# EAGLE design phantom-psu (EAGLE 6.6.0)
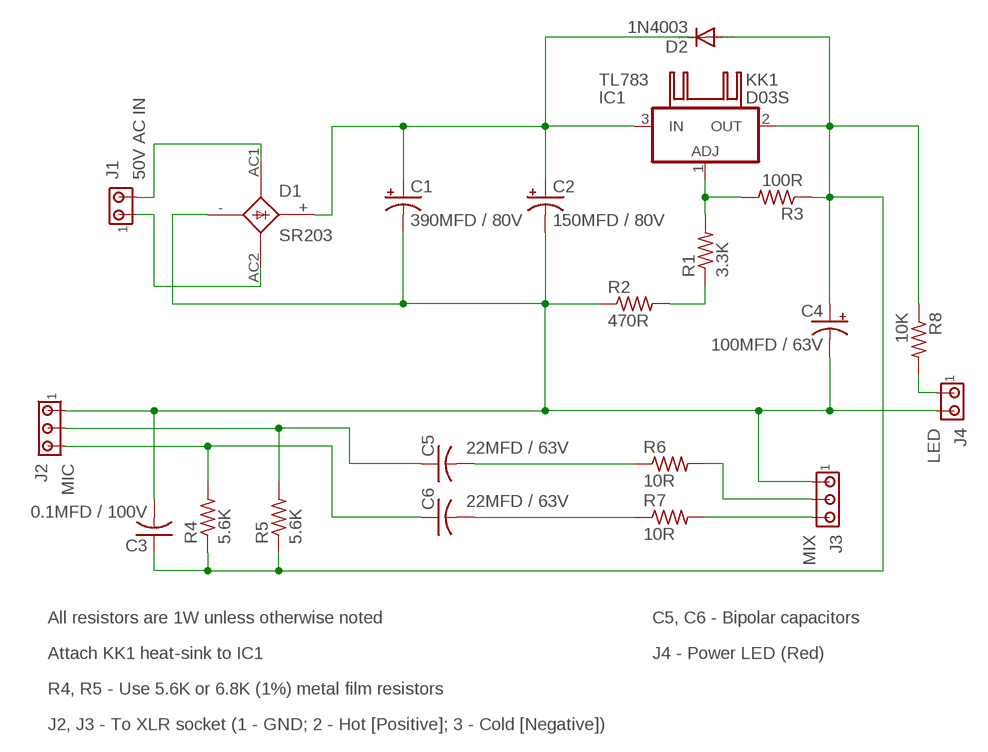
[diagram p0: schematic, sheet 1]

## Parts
C1  390MFD / 80V  CPOL-USE5-10.5  [E5-10,5]
C2  150MFD / 80V  CPOL-USE5-10.5  [E5-10,5]
C3  0.1MFD / 100V  C-US075-063X106  [C075-063X106]
C4  100MFD / 63V  CPOL-USE3.5-8  [E3,5-8]
C5  22MFD / 63V  NON-POL_CAP  [CAP]
C6  22MFD / 63V  NON-POL_CAP  [CAP]
D1  SR203  RS203  [RS-2]
D2  1N4003  1N4004  [DO41-10]
IC1  TL783  [TO220V]
J1  50V AC IN  MTA02-156  [1X2MTA]
J2  MIC  350760-4  [350760-4]
J3  MIX  350760-4  [350760-4]
J4  LED  MTA02-100  [10X02MTA]
KK1  D03S  [D03S]
R1  3.3K  R-US_0207/12  [0207/12]
R2  470R  R-US_0207/12  [0207/12]
R3  100R  R-US_0207/12  [0207/12]
R4  5.6K  R-US_0207/12  [0207/12]
R5  5.6K  R-US_0207/12  [0207/12]
R6  10R  R-US_0207/12  [0207/12]
R7  10R  R-US_0207/12  [0207/12]
R8  10K  R-US_0207/12  [0207/12]

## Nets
48V: C3.1 C4.+ D2.A IC1.2(OUT) R3.1 R4.1 R5.1 R8.1
GND: C1.- C2.- C3.2 C4.- D1.-(GND) J2.1 J3.1 J4.2 R2.1
N$1: D1.AC1 J1.2
N$2: D1.AC2 J1.1
N$3: J3.3 R7.2
N$4: C1.+ C2.+ D1.+ D2.C IC1.3(IN)
N$5: R1.1 R2.2
N$6: J3.2 R6.2
N$7: IC1.1(ADJ) R1.2 R3.2
N$8: C5.- R6.1
N$9: C6.+ J2.3 R4.2
N$10: C5.+ J2.2 R5.2
N$11: C6.- R7.1
N$12: J4.1 R8.2

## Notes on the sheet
- All resistors are 1W unless otherwise noted | C5, C6 - Bipolar capacitors
- Attach KK1 heat-sink to IC1 | J4 - Power LED (Red)
- R4, R5 - Use 5.6K or 6.8K (1%) metal film resistors
- J2, J3 - To XLR socket (1 - GND; 2 - Hot [Positive]; 3 - Cold [Negative])

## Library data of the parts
C1 C2 C4 = rcl:CPOL-US: POLARIZED CAPACITOR, American symbol
C3 = resistor:C-US: CAPACITOR, American symbol
C5 C6 = phantom-psu:NON-POL_CAP: Non polar capaictor
D1 = phantom-psu:RS203: Single phase 2.0A bridge rectifier
D2 = diode:1N4004: DIODE
IC1 = phantom-psu:TL783: High-voltage adjustable regulator
J1 = con-amp:MTA02-156: AMP connector
J2 J3 = con-amp:350760-4: Universal MATE-N-LOK .250" Centerline, 600 V, 19 - 36 A max Source: http://catalog.tycoelectronics.com/ .. ENG_CD_350760_T.pdf
J4 = con-amp:MTA02-100: AMP connector
KK1 = heatsink:D03S: HEATSINK
R1-R8 = resistor:R-US_: RESISTOR, American symbol

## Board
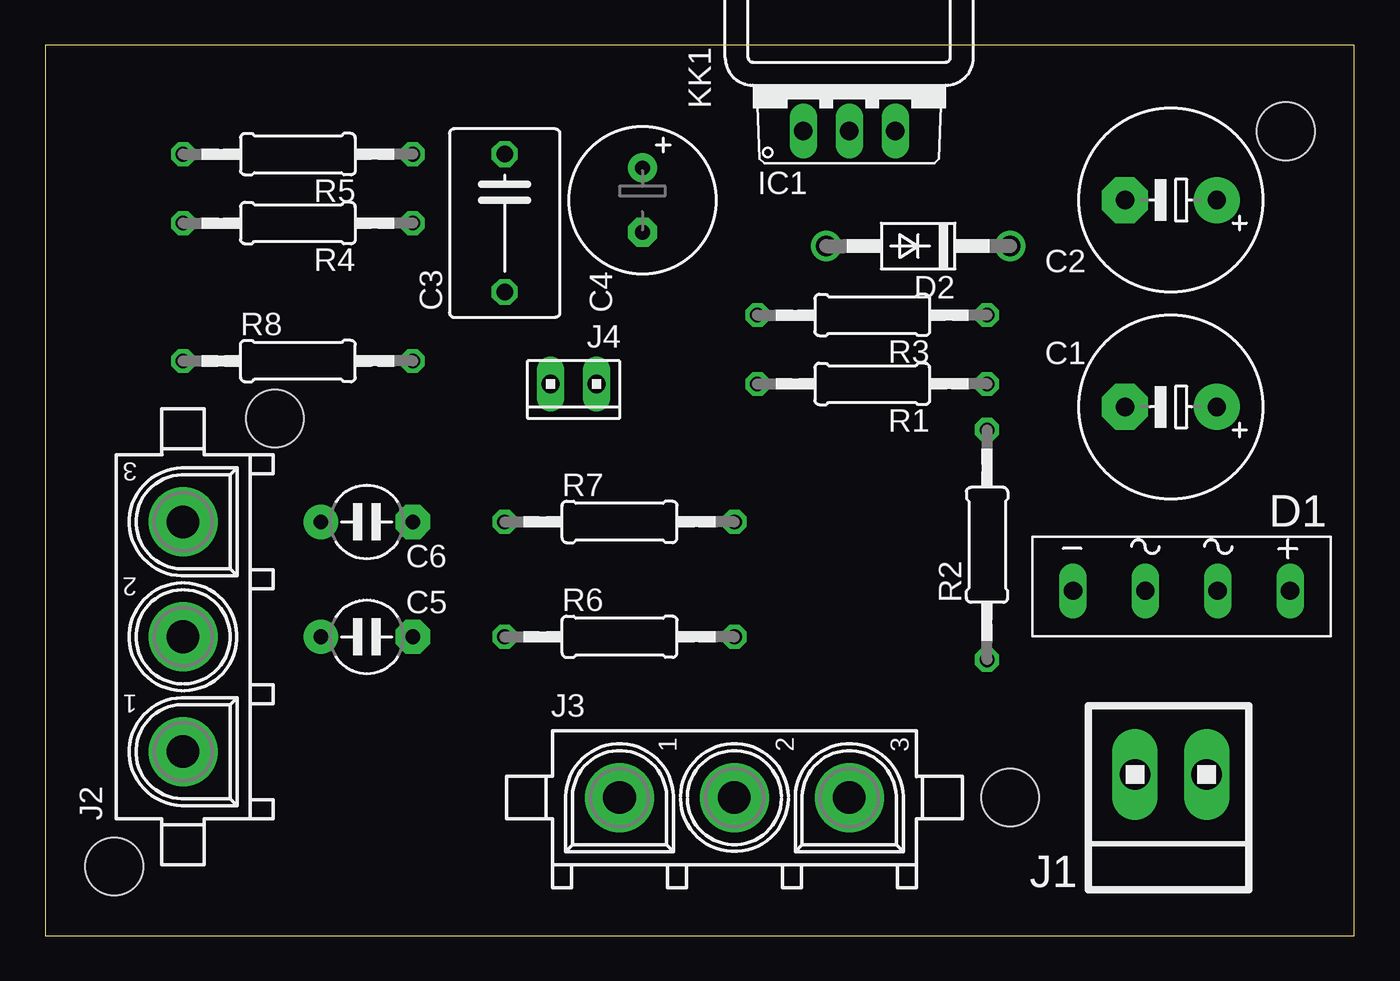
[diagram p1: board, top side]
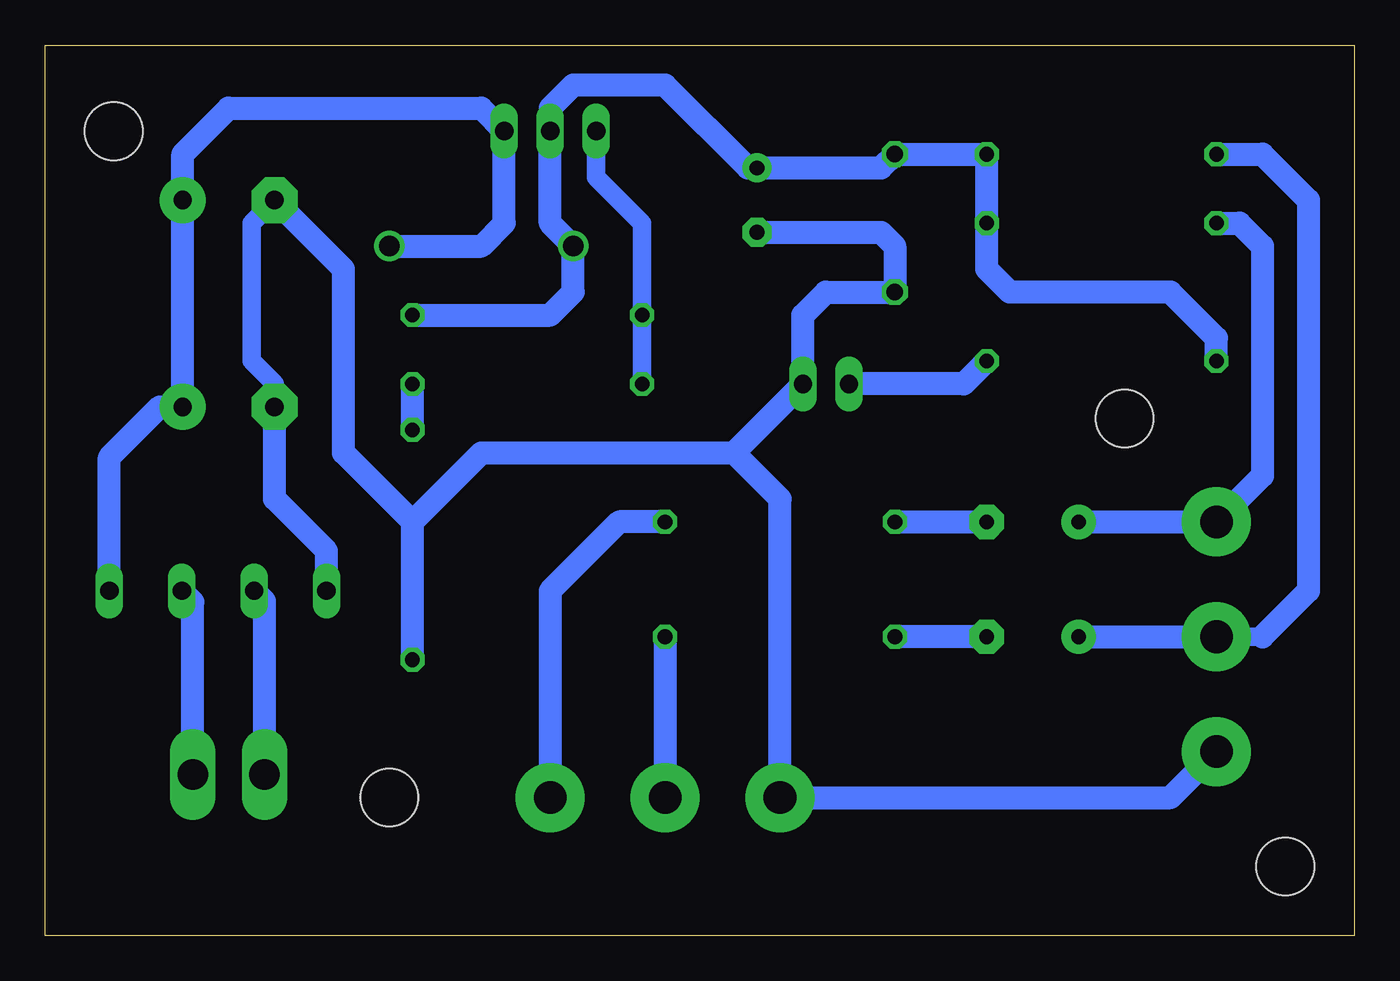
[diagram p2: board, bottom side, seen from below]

Size 72.37 x 49.2 mm. Coordinates in mm from the lower left corner, seen from the top.
Outline: 0,0 72.37,0 72.37,49.2 0,49.2 0,0
Copper layers (1*16): Top 0.035mm / dielectric 1.5mm / Bottom 0.035mm
Design rules "default": minimum track width 10mil, minimum drill 24mil, track to track 8mil, track to pad 8mil, pad to pad 8mil, via to via 8mil, smd to smd 8mil, copper to edge 40mil, drill to drill 8mil, minimum pad ring 10mil, minimum via ring 8mil, stop-mask expansion 4mil, vias tented up to drill 0mil, thermal gap 10mil
Holes 3.2 mm at 53.34,7.62 12.7,28.58 3.81,3.81 68.58,44.45

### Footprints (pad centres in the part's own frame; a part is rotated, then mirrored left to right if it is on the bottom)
E5-10,5 = drill 1.016 pad 2.54: + -2.54,0 | drill 1.016 pad 2.54 octagon: - 2.54,0
C075-063X106 = drill 0.914 octagon: 1 -3.81,0; 2 3.81,0
E3,5-8 = drill 0.813 pad 1.6: + -1.778,0 | drill 0.813 pad 1.6 octagon: - 1.778,0
CAP = drill 0.813 pad 1.905: + -2.54,0 | drill 0.813 pad 1.905 octagon: - 2.54,0
RS-2 = drill 1.016 long: + -0.24,0; - 11.76,0; AC1 3.76,0; AC2 7.76,0
DO41-10 = drill 1.118: A 5.08,0; C -5.08,0
TO220V = drill 1.016 long: 1 -2.54,0; 2 0,0; 3 2.54,0
1X2MTA = drill 1.676 long: 1 1.981,0; 2 -1.981,0
350760-4 = drill 1.8 pad 3.81: 1 -6.35,0; 2 0,0; 3 6.35,0
10X02MTA = drill 1.016 long: 1 1.27,0; 2 -1.27,0
0207/12 = drill 0.813 octagon: 1 -6.35,0; 2 6.35,0

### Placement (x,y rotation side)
C1  62.23,29.21 180 top
C2  62.23,40.64 180 top
C3  25.4,39.37 270 top
C4  33.02,40.64 270 top
C5  17.78,16.51 0 top
C6  17.78,22.86 0 top
D1  68.58,19.05 180 top
D2  48.26,38.1 180 top
IC1  44.45,44.45 0 top
J1  62.23,8.89 180 top
J2  7.62,16.51 90 top
J3  38.1,7.62 0 top
J4  29.21,30.48 180 top
KK1  44.45,48.26 0 top
R1  45.72,30.48 180 top
R2  52.07,21.59 90 top
R3  45.72,34.29 180 top
R4  13.97,39.37 180 top
R5  13.97,43.18 180 top
R6  31.75,16.51 0 top
R7  31.75,22.86 0 top
R8  13.97,31.75 0 top

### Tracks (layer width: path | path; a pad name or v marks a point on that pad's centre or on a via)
48V
  Bottom 1.016: 44.45,45.72 IC1.2
  Bottom 1.27: R3.1 44.45,34.29 43.18,35.56 D2.A 44.45,39.37 IC1.2 | 44.45,45.72 43.18,46.99 38.1,46.99 33.53,42.42 C4.+ 26.16,42.42 C3.1 R5.1 R4.1 20.32,36.83 19.05,35.56 10.16,35.56 7.62,33.02 R8.1
GND
  Bottom 1.016: C1.- 59.69,30.48 60.96,31.75 60.96,39.37 C2.-
  Bottom 1.27: D1.- 56.82,21.26 59.69,24.13 C1.- | R2.1 52.07,22.86 | 52.07,22.86 55.88,26.67 55.88,36.83 C2.- | 52.07,22.86 48.26,26.67 34.29,26.67 | 34.29,26.67 J4.2 30.48,34.29 29.21,35.56 C3.2 25.4,38.1 26.16,38.86 C4.- | J2.1 10.16,7.62 J3.1 31.75,24.13 34.29,26.67
N$1
  Bottom 1.27: J1.2 64.21,18.44 D1.AC1
N$2
  Bottom 1.27: J1.1 60.25,18.48 D1.AC2
N$3
  Bottom 1.27: R7.2 40.64,22.86 44.45,19.05 J3.3
N$4
  Bottom 1.27: D1.+ 68.82,26.43 66.04,29.21 C1.+ C2.+ 64.77,43.18 62.23,45.72 48.26,45.72 IC1.3 46.99,39.37 48.26,38.1 D2.C
N$5
  Bottom 1.27: R2.2 R1.1
N$6
  Bottom 1.27: R6.2 J3.2
N$7
  Bottom 1.016: R1.2 R3.2 39.37,39.37 41.91,41.91 IC1.1
N$8
  Bottom 1.27: C5.- R6.1
N$9
  Bottom 1.27: C6.+ J2.3 5.08,25.4 5.08,38.1 6.35,39.37 R4.2
N$10
  Bottom 1.016: 5.08,16.51 J2.2
  Bottom 1.27: C5.+ J2.2 | R5.2 5.08,43.18 2.54,40.64 2.54,19.05 5.08,16.51
N$11
  Bottom 1.27: R7.1 C6.-
N$12
  Bottom 1.27: R8.2 21.59,30.48 J4.1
